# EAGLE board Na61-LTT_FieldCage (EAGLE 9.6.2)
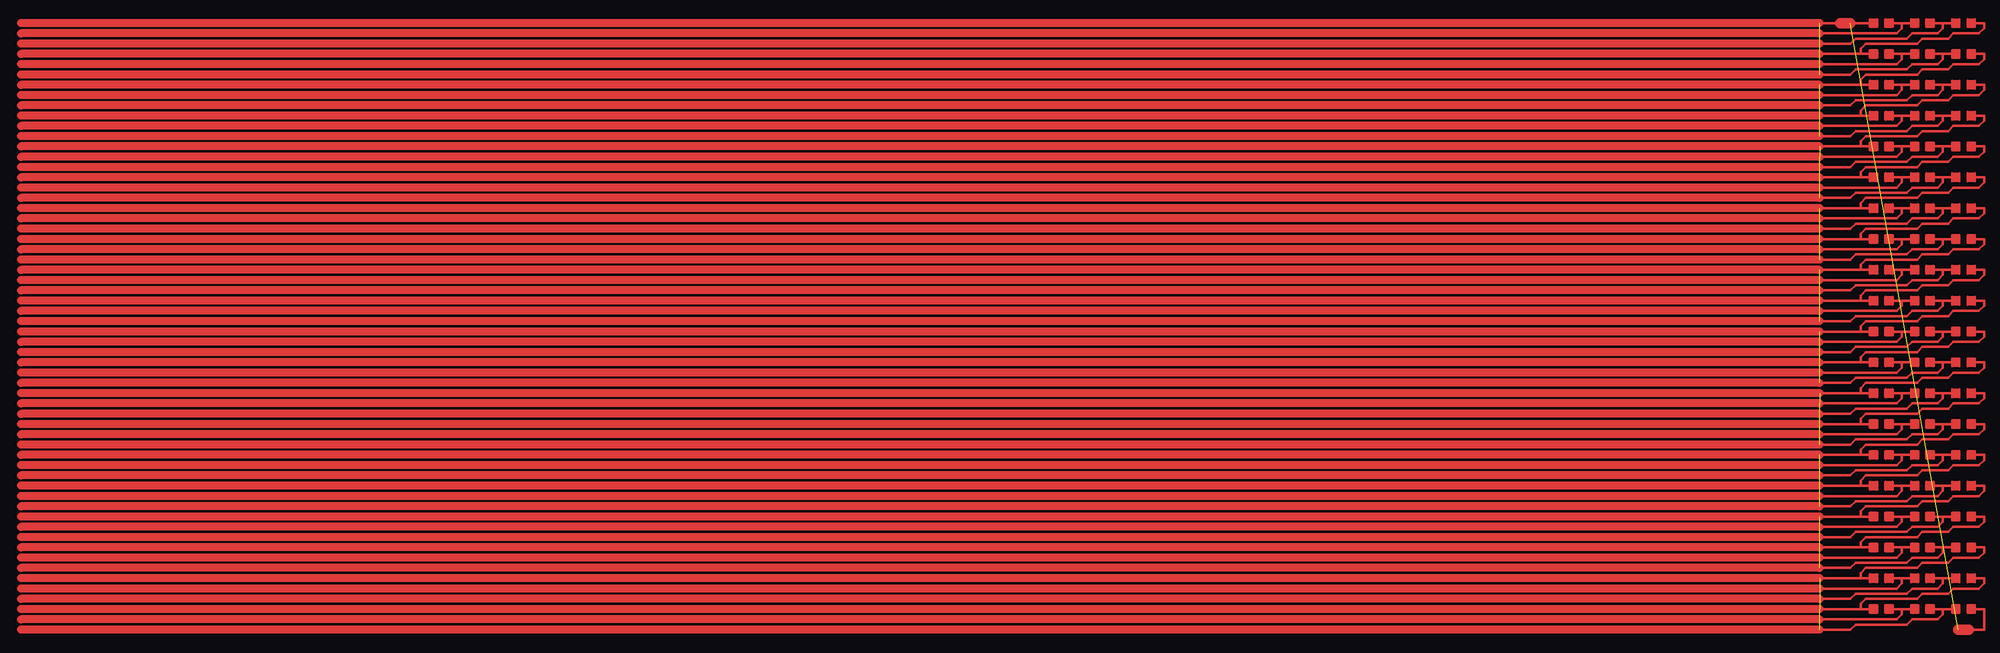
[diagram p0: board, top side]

No outline drawn. Coordinates in mm, seen from the top.
Copper layers (1*16): Top 0.035mm / dielectric 1.5mm / Bottom 0.035mm
Design rules "default": minimum track width 10mil, minimum drill 24mil, track to track 8mil, track to pad 8mil, pad to pad 8mil, via to via 8mil, smd to smd 8mil, copper to edge 40mil, drill to drill 8mil, minimum pad ring 10mil, minimum via ring 8mil, stop-mask expansion 4mil, vias tented up to drill 0mil, thermal gap 10mil

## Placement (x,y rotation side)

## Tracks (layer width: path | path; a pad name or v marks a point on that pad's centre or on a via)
S$1  (5 unrouted)
  Top 1.6: 0,2 -350,2 | 0,4 -350,4 | 0,6 -350,6 | 0,8 -350,8 | 0,10 -350,10 | 0,12 -350,12
S$2
  Top 0.406: 9.8,23.2 9.8,24.8 11.2,24.8 11.2,23.2 9.8,23.2
S$3
  Top 0.406: 12.8,23.2 12.8,24.8 14.2,24.8 14.2,23.2 12.8,23.2
S$4
  Top 0.406: 17.8,23.2 17.8,24.8 19.2,24.8 19.2,23.2 17.8,23.2
S$5
  Top 0.406: 20.8,23.2 20.8,24.8 22.2,24.8 22.2,23.2 20.8,23.2
S$6
  Top 0.406: 25.8,23.2 25.8,24.8 27.2,24.8 27.2,23.2 25.8,23.2
S$7
  Top 0.406: 28.8,23.2 28.8,24.8 30.2,24.8 30.2,23.2 28.8,23.2
S$8
  Top 0.508: 10,24 0,24
S$9
  Top 0.508: 14,24 16,24 | 16,24 18,24 | 16,24 16,23 15,22 0,22
S$10
  Top 0.508: 22,24 24,24 | 24,24 26,24 | 24,24 24,23 23,22 18,22 17,21 7,21 6,20 0,20
S$11
  Top 0.508: 8,18 8,19 9,20 19,20 20,21 25,21 26,22 31,22 32,23 32,24 30,24
S$12
  Top 0.406: 9.8,17.2 9.8,18.8 11.2,18.8 11.2,17.2 9.8,17.2
S$13
  Top 0.406: 12.8,17.2 12.8,18.8 14.2,18.8 14.2,17.2 12.8,17.2
S$14
  Top 0.406: 17.8,17.2 17.8,18.8 19.2,18.8 19.2,17.2 17.8,17.2
S$15
  Top 0.406: 9.8,5.2 9.8,6.8 11.2,6.8 11.2,5.2 9.8,5.2
S$16
  Top 0.406: 9.8,11.2 9.8,12.8 11.2,12.8 11.2,11.2 9.8,11.2
S$17
  Top 0.406: 12.8,11.2 12.8,12.8 14.2,12.8 14.2,11.2 12.8,11.2
S$18
  Top 0.406: 12.8,5.2 12.8,6.8 14.2,6.8 14.2,5.2 12.8,5.2
S$19
  Top 0.406: 17.8,11.2 17.8,12.8 19.2,12.8 19.2,11.2 17.8,11.2
S$20
  Top 0.406: 20.8,11.2 20.8,12.8 22.2,12.8 22.2,11.2 20.8,11.2
S$21
  Top 0.406: 25.8,11.2 25.8,12.8 27.2,12.8 27.2,11.2 25.8,11.2
S$22
  Top 0.406: 28.8,11.2 28.8,12.8 30.2,12.8 30.2,11.2 28.8,11.2
S$23
  Top 0.508: 8,6 8,7 9,8 19,8 20,9 25,9 26,10 31,10 32,11 32,12 30,12
S$24
  Top 0.406: 17.8,5.2 17.8,6.8 19.2,6.8 19.2,5.2 17.8,5.2
S$25
  Top 0.406: 20.8,5.2 20.8,6.8 22.2,6.8 22.2,5.2 20.8,5.2
S$26
  Top 0.508: 10,12 0,12
S$27
  Top 0.508: 14,12 16,12 | 16,12 18,12 | 16,12 16,11 15,10 0,10
S$28
  Top 0.508: 22,12 24,12 | 24,12 26,12 | 24,12 24,11 23,10 18,10 17,9 7,9 6,8 0,8
S$29
  Top 0.406: 25.8,5.2 25.8,6.8 27.2,6.8 27.2,5.2 25.8,5.2
S$30
  Top 0.406: 28.8,5.2 28.8,6.8 30.2,6.8 30.2,5.2 28.8,5.2
S$31
  Top 0.508: 10,6 0,6
S$32
  Top 0.508: 14,6 16,6 | 16,6 18,6 | 16,6 16,5 15,4 0,4
S$33
  Top 0.508: 22,6 24,6 | 24,6 26,6 | 24,6 24,5 23,4 18,4 17,3 7,3 6,2 0,2
S$34
  Top 0.508: 29,2 32,2 32,6 30,6
S$35
  Top 0.406: 20.8,17.2 20.8,18.8 22.2,18.8 22.2,17.2 20.8,17.2
S$36
  Top 0.406: 25.8,17.2 25.8,18.8 27.2,18.8 27.2,17.2 25.8,17.2
S$37
  Top 0.406: 28.8,17.2 28.8,18.8 30.2,18.8 30.2,17.2 28.8,17.2
S$38
  Top 0.508: 10,18 0,18
S$39
  Top 0.508: 14,18 16,18 | 16,18 18,18 | 16,18 16,17 15,16 0,16
S$40
  Top 0.508: 22,18 24,18 | 24,18 26,18 | 24,18 24,17 23,16 18,16 17,15 7,15 6,14 0,14
S$41
  Top 0.508: 8,12 8,13 9,14 19,14 20,15 25,15 26,16 31,16 32,17 32,18 30,18
S$42  (5 unrouted)
  Top 1.6: 0,14 -350,14 | 0,16 -350,16 | 0,18 -350,18 | 0,20 -350,20 | 0,22 -350,22 | 0,24 -350,24
S$43
  Top 0.406: 9.8,35.2 9.8,36.8 11.2,36.8 11.2,35.2 9.8,35.2
S$44
  Top 0.406: 12.8,35.2 12.8,36.8 14.2,36.8 14.2,35.2 12.8,35.2
S$45
  Top 0.406: 17.8,35.2 17.8,36.8 19.2,36.8 19.2,35.2 17.8,35.2
S$46
  Top 0.406: 20.8,35.2 20.8,36.8 22.2,36.8 22.2,35.2 20.8,35.2
S$47
  Top 0.406: 25.8,35.2 25.8,36.8 27.2,36.8 27.2,35.2 25.8,35.2
S$48
  Top 0.406: 28.8,35.2 28.8,36.8 30.2,36.8 30.2,35.2 28.8,35.2
S$49
  Top 0.508: 10,36 0,36
S$50
  Top 0.508: 14,36 16,36 | 16,36 18,36 | 16,36 16,35 15,34 0,34
S$51
  Top 0.508: 22,36 24,36 | 24,36 26,36 | 24,36 24,35 23,34 18,34 17,33 7,33 6,32 0,32
S$52
  Top 0.508: 8,30 8,31 9,32 19,32 20,33 25,33 26,34 31,34 32,35 32,36 30,36
S$53
  Top 0.406: 9.8,29.2 9.8,30.8 11.2,30.8 11.2,29.2 9.8,29.2
S$54
  Top 0.406: 12.8,29.2 12.8,30.8 14.2,30.8 14.2,29.2 12.8,29.2
S$55
  Top 0.406: 17.8,29.2 17.8,30.8 19.2,30.8 19.2,29.2 17.8,29.2
S$56
  Top 0.406: 20.8,29.2 20.8,30.8 22.2,30.8 22.2,29.2 20.8,29.2
S$57
  Top 0.406: 25.8,29.2 25.8,30.8 27.2,30.8 27.2,29.2 25.8,29.2
S$58
  Top 0.406: 28.8,29.2 28.8,30.8 30.2,30.8 30.2,29.2 28.8,29.2
S$59
  Top 0.508: 10,30 0,30
S$60
  Top 0.508: 14,30 16,30 | 16,30 18,30 | 16,30 16,29 15,28 0,28
S$61
  Top 0.508: 22,30 24,30 | 24,30 26,30 | 24,30 24,29 23,28 18,28 17,27 7,27 6,26 0,26
S$62
  Top 0.508: 8,24 8,25 9,26 19,26 20,27 25,27 26,28 31,28 32,29 32,30 30,30
S$63  (5 unrouted)
  Top 1.6: 0,26 -350,26 | 0,28 -350,28 | 0,30 -350,30 | 0,32 -350,32 | 0,34 -350,34 | 0,36 -350,36
S$64
  Top 0.406: 9.8,47.2 9.8,48.8 11.2,48.8 11.2,47.2 9.8,47.2
S$65
  Top 0.406: 12.8,47.2 12.8,48.8 14.2,48.8 14.2,47.2 12.8,47.2
S$66
  Top 0.406: 17.8,47.2 17.8,48.8 19.2,48.8 19.2,47.2 17.8,47.2
S$67
  Top 0.406: 20.8,47.2 20.8,48.8 22.2,48.8 22.2,47.2 20.8,47.2
S$68
  Top 0.406: 25.8,47.2 25.8,48.8 27.2,48.8 27.2,47.2 25.8,47.2
S$69
  Top 0.406: 28.8,47.2 28.8,48.8 30.2,48.8 30.2,47.2 28.8,47.2
S$70
  Top 0.508: 10,48 0,48
S$71
  Top 0.508: 14,48 16,48 | 16,48 18,48 | 16,48 16,47 15,46 0,46
S$72
  Top 0.508: 22,48 24,48 | 24,48 26,48 | 24,48 24,47 23,46 18,46 17,45 7,45 6,44 0,44
S$73
  Top 0.508: 8,42 8,43 9,44 19,44 20,45 25,45 26,46 31,46 32,47 32,48 30,48
S$74
  Top 0.406: 9.8,41.2 9.8,42.8 11.2,42.8 11.2,41.2 9.8,41.2
S$75
  Top 0.406: 12.8,41.2 12.8,42.8 14.2,42.8 14.2,41.2 12.8,41.2
S$76
  Top 0.406: 17.8,41.2 17.8,42.8 19.2,42.8 19.2,41.2 17.8,41.2
S$77
  Top 0.406: 20.8,41.2 20.8,42.8 22.2,42.8 22.2,41.2 20.8,41.2
S$78
  Top 0.406: 25.8,41.2 25.8,42.8 27.2,42.8 27.2,41.2 25.8,41.2
S$79
  Top 0.406: 28.8,41.2 28.8,42.8 30.2,42.8 30.2,41.2 28.8,41.2
S$80
  Top 0.508: 10,42 0,42
S$81
  Top 0.508: 14,42 16,42 | 16,42 18,42 | 16,42 16,41 15,40 0,40
S$82
  Top 0.508: 22,42 24,42 | 24,42 26,42 | 24,42 24,41 23,40 18,40 17,39 7,39 6,38 0,38
S$83
  Top 0.508: 8,36 8,37 9,38 19,38 20,39 25,39 26,40 31,40 32,41 32,42 30,42
S$84  (5 unrouted)
  Top 1.6: 0,38 -350,38 | 0,40 -350,40 | 0,42 -350,42 | 0,44 -350,44 | 0,46 -350,46 | 0,48 -350,48
S$85
  Top 0.406: 9.8,59.2 9.8,60.8 11.2,60.8 11.2,59.2 9.8,59.2
S$86
  Top 0.406: 12.8,59.2 12.8,60.8 14.2,60.8 14.2,59.2 12.8,59.2
S$87
  Top 0.406: 17.8,59.2 17.8,60.8 19.2,60.8 19.2,59.2 17.8,59.2
S$88
  Top 0.406: 20.8,59.2 20.8,60.8 22.2,60.8 22.2,59.2 20.8,59.2
S$89
  Top 0.406: 25.8,59.2 25.8,60.8 27.2,60.8 27.2,59.2 25.8,59.2
S$90
  Top 0.406: 28.8,59.2 28.8,60.8 30.2,60.8 30.2,59.2 28.8,59.2
S$91
  Top 0.508: 10,60 0,60
S$92
  Top 0.508: 14,60 16,60 | 16,60 18,60 | 16,60 16,59 15,58 0,58
S$93
  Top 0.508: 22,60 24,60 | 24,60 26,60 | 24,60 24,59 23,58 18,58 17,57 7,57 6,56 0,56
S$94
  Top 0.508: 8,54 8,55 9,56 19,56 20,57 25,57 26,58 31,58 32,59 32,60 30,60
S$95
  Top 0.406: 9.8,53.2 9.8,54.8 11.2,54.8 11.2,53.2 9.8,53.2
S$96
  Top 0.406: 12.8,53.2 12.8,54.8 14.2,54.8 14.2,53.2 12.8,53.2
S$97
  Top 0.406: 17.8,53.2 17.8,54.8 19.2,54.8 19.2,53.2 17.8,53.2
S$98
  Top 0.406: 20.8,53.2 20.8,54.8 22.2,54.8 22.2,53.2 20.8,53.2
S$99
  Top 0.406: 25.8,53.2 25.8,54.8 27.2,54.8 27.2,53.2 25.8,53.2
S$100
  Top 0.406: 28.8,53.2 28.8,54.8 30.2,54.8 30.2,53.2 28.8,53.2
S$101
  Top 0.508: 10,54 0,54
S$102
  Top 0.508: 14,54 16,54 | 16,54 18,54 | 16,54 16,53 15,52 0,52
S$103
  Top 0.508: 22,54 24,54 | 24,54 26,54 | 24,54 24,53 23,52 18,52 17,51 7,51 6,50 0,50
S$104
  Top 0.508: 8,48 8,49 9,50 19,50 20,51 25,51 26,52 31,52 32,53 32,54 30,54
S$105  (5 unrouted)
  Top 1.6: 0,50 -350,50 | 0,52 -350,52 | 0,54 -350,54 | 0,56 -350,56 | 0,58 -350,58 | 0,60 -350,60
S$106
  Top 0.406: 9.8,71.2 9.8,72.8 11.2,72.8 11.2,71.2 9.8,71.2
S$107
  Top 0.406: 12.8,71.2 12.8,72.8 14.2,72.8 14.2,71.2 12.8,71.2
S$108
  Top 0.406: 17.8,71.2 17.8,72.8 19.2,72.8 19.2,71.2 17.8,71.2
S$109
  Top 0.406: 20.8,71.2 20.8,72.8 22.2,72.8 22.2,71.2 20.8,71.2
S$110
  Top 0.406: 25.8,71.2 25.8,72.8 27.2,72.8 27.2,71.2 25.8,71.2
S$111
  Top 0.406: 28.8,71.2 28.8,72.8 30.2,72.8 30.2,71.2 28.8,71.2
S$112
  Top 0.508: 10,72 0,72
S$113
  Top 0.508: 14,72 16,72 | 16,72 18,72 | 16,72 16,71 15,70 0,70
S$114
  Top 0.508: 22,72 24,72 | 24,72 26,72 | 24,72 24,71 23,70 18,70 17,69 7,69 6,68 0,68
S$115
  Top 0.508: 8,66 8,67 9,68 19,68 20,69 25,69 26,70 31,70 32,71 32,72 30,72
S$116
  Top 0.406: 9.8,65.2 9.8,66.8 11.2,66.8 11.2,65.2 9.8,65.2
S$117
  Top 0.406: 12.8,65.2 12.8,66.8 14.2,66.8 14.2,65.2 12.8,65.2
S$118
  Top 0.406: 17.8,65.2 17.8,66.8 19.2,66.8 19.2,65.2 17.8,65.2
S$119
  Top 0.406: 20.8,65.2 20.8,66.8 22.2,66.8 22.2,65.2 20.8,65.2
S$120
  Top 0.406: 25.8,65.2 25.8,66.8 27.2,66.8 27.2,65.2 25.8,65.2
S$121
  Top 0.406: 28.8,65.2 28.8,66.8 30.2,66.8 30.2,65.2 28.8,65.2
S$122
  Top 0.508: 10,66 0,66
S$123
  Top 0.508: 14,66 16,66 | 16,66 18,66 | 16,66 16,65 15,64 0,64
S$124
  Top 0.508: 22,66 24,66 | 24,66 26,66 | 24,66 24,65 23,64 18,64 17,63 7,63 6,62 0,62
S$125
  Top 0.508: 8,60 8,61 9,62 19,62 20,63 25,63 26,64 31,64 32,65 32,66 30,66
S$126  (5 unrouted)
  Top 1.6: 0,62 -350,62 | 0,64 -350,64 | 0,66 -350,66 | 0,68 -350,68 | 0,70 -350,70 | 0,72 -350,72
S$127
  Top 0.406: 9.8,83.2 9.8,84.8 11.2,84.8 11.2,83.2 9.8,83.2
S$128
  Top 0.406: 12.8,83.2 12.8,84.8 14.2,84.8 14.2,83.2 12.8,83.2
S$129
  Top 0.406: 17.8,83.2 17.8,84.8 19.2,84.8 19.2,83.2 17.8,83.2
S$130
  Top 0.406: 20.8,83.2 20.8,84.8 22.2,84.8 22.2,83.2 20.8,83.2
S$131
  Top 0.406: 25.8,83.2 25.8,84.8 27.2,84.8 27.2,83.2 25.8,83.2
S$132
  Top 0.406: 28.8,83.2 28.8,84.8 30.2,84.8 30.2,83.2 28.8,83.2
S$133
  Top 0.508: 10,84 0,84
S$134
  Top 0.508: 14,84 16,84 | 16,84 18,84 | 16,84 16,83 15,82 0,82
S$135
  Top 0.508: 22,84 24,84 | 24,84 26,84 | 24,84 24,83 23,82 18,82 17,81 7,81 6,80 0,80
S$136
  Top 0.508: 8,78 8,79 9,80 19,80 20,81 25,81 26,82 31,82 32,83 32,84 30,84
S$137
  Top 0.406: 9.8,77.2 9.8,78.8 11.2,78.8 11.2,77.2 9.8,77.2
S$138
  Top 0.406: 12.8,77.2 12.8,78.8 14.2,78.8 14.2,77.2 12.8,77.2
S$139
  Top 0.406: 17.8,77.2 17.8,78.8 19.2,78.8 19.2,77.2 17.8,77.2
S$140
  Top 0.406: 20.8,77.2 20.8,78.8 22.2,78.8 22.2,77.2 20.8,77.2
S$141
  Top 0.406: 25.8,77.2 25.8,78.8 27.2,78.8 27.2,77.2 25.8,77.2
S$142
  Top 0.406: 28.8,77.2 28.8,78.8 30.2,78.8 30.2,77.2 28.8,77.2
S$143
  Top 0.508: 10,78 0,78
S$144
  Top 0.508: 14,78 16,78 | 16,78 18,78 | 16,78 16,77 15,76 0,76
S$145
  Top 0.508: 22,78 24,78 | 24,78 26,78 | 24,78 24,77 23,76 18,76 17,75 7,75 6,74 0,74
S$146
  Top 0.508: 8,72 8,73 9,74 19,74 20,75 25,75 26,76 31,76 32,77 32,78 30,78
S$147  (5 unrouted)
  Top 1.6: 0,74 -350,74 | 0,76 -350,76 | 0,78 -350,78 | 0,80 -350,80 | 0,82 -350,82 | 0,84 -350,84
S$148
  Top 0.406: 9.8,95.2 9.8,96.8 11.2,96.8 11.2,95.2 9.8,95.2
S$149
  Top 0.406: 12.8,95.2 12.8,96.8 14.2,96.8 14.2,95.2 12.8,95.2
S$150
  Top 0.406: 17.8,95.2 17.8,96.8 19.2,96.8 19.2,95.2 17.8,95.2
S$151
  Top 0.406: 20.8,95.2 20.8,96.8 22.2,96.8 22.2,95.2 20.8,95.2
S$152
  Top 0.406: 25.8,95.2 25.8,96.8 27.2,96.8 27.2,95.2 25.8,95.2
S$153
  Top 0.406: 28.8,95.2 28.8,96.8 30.2,96.8 30.2,95.2 28.8,95.2
S$154
  Top 0.508: 10,96 0,96
S$155
  Top 0.508: 14,96 16,96 | 16,96 18,96 | 16,96 16,95 15,94 0,94
S$156
  Top 0.508: 22,96 24,96 | 24,96 26,96 | 24,96 24,95 23,94 18,94 17,93 7,93 6,92 0,92
S$157
  Top 0.508: 8,90 8,91 9,92 19,92 20,93 25,93 26,94 31,94 32,95 32,96 30,96
S$158
  Top 0.406: 9.8,89.2 9.8,90.8 11.2,90.8 11.2,89.2 9.8,89.2
S$159
  Top 0.406: 12.8,89.2 12.8,90.8 14.2,90.8 14.2,89.2 12.8,89.2
S$160
  Top 0.406: 17.8,89.2 17.8,90.8 19.2,90.8 19.2,89.2 17.8,89.2
S$161
  Top 0.406: 20.8,89.2 20.8,90.8 22.2,90.8 22.2,89.2 20.8,89.2
S$162
  Top 0.406: 25.8,89.2 25.8,90.8 27.2,90.8 27.2,89.2 25.8,89.2
S$163
  Top 0.406: 28.8,89.2 28.8,90.8 30.2,90.8 30.2,89.2 28.8,89.2
S$164
  Top 0.508: 10,90 0,90
S$165
  Top 0.508: 14,90 16,90 | 16,90 18,90 | 16,90 16,89 15,88 0,88
S$166
  Top 0.508: 22,90 24,90 | 24,90 26,90 | 24,90 24,89 23,88 18,88 17,87 7,87 6,86 0,86
S$167
  Top 0.508: 8,84 8,85 9,86 19,86 20,87 25,87 26,88 31,88 32,89 32,90 30,90
S$168  (5 unrouted)
  Top 1.6: 0,86 -350,86 | 0,88 -350,88 | 0,90 -350,90 | 0,92 -350,92 | 0,94 -350,94 | 0,96 -350,96
S$169
  Top 0.406: 9.8,107.2 9.8,108.8 11.2,108.8 11.2,107.2 9.8,107.2
S$170
  Top 0.406: 12.8,107.2 12.8,108.8 14.2,108.8 14.2,107.2 12.8,107.2
S$171
  Top 0.406: 17.8,107.2 17.8,108.8 19.2,108.8 19.2,107.2 17.8,107.2
S$172
  Top 0.406: 20.8,107.2 20.8,108.8 22.2,108.8 22.2,107.2 20.8,107.2
S$173
  Top 0.406: 25.8,107.2 25.8,108.8 27.2,108.8 27.2,107.2 25.8,107.2
S$174
  Top 0.406: 28.8,107.2 28.8,108.8 30.2,108.8 30.2,107.2 28.8,107.2
S$175
  Top 0.508: 10,108 0,108
S$176
  Top 0.508: 14,108 16,108 | 16,108 18,108 | 16,108 16,107 15,106 0,106
S$177
  Top 0.508: 22,108 24,108 | 24,108 26,108 | 24,108 24,107 23,106 18,106 17,105 7,105 6,104 0,104
S$178
  Top 0.508: 8,102 8,103 9,104 19,104 20,105 25,105 26,106 31,106 32,107 32,108 30,108
S$179
  Top 0.406: 9.8,101.2 9.8,102.8 11.2,102.8 11.2,101.2 9.8,101.2
S$180
  Top 0.406: 12.8,101.2 12.8,102.8 14.2,102.8 14.2,101.2 12.8,101.2
S$181
  Top 0.406: 17.8,101.2 17.8,102.8 19.2,102.8 19.2,101.2 17.8,101.2
S$182
  Top 0.406: 20.8,101.2 20.8,102.8 22.2,102.8 22.2,101.2 20.8,101.2
S$183
  Top 0.406: 25.8,101.2 25.8,102.8 27.2,102.8 27.2,101.2 25.8,101.2
S$184
  Top 0.406: 28.8,101.2 28.8,102.8 30.2,102.8 30.2,101.2 28.8,101.2
S$185
  Top 0.508: 10,102 0,102
S$186
  Top 0.508: 14,102 16,102 | 16,102 18,102 | 16,102 16,101 15,100 0,100
S$187
  Top 0.508: 22,102 24,102 | 24,102 26,102 | 24,102 24,101 23,100 18,100 17,99 7,99 6,98 0,98
S$188
  Top 0.508: 8,96 8,97 9,98 19,98 20,99 25,99 26,100 31,100 32,101 32,102 30,102
S$189  (5 unrouted)
  Top 1.6: 0,98 -350,98 | 0,100 -350,100 | 0,102 -350,102 | 0,104 -350,104 | 0,106 -350,106 | 0,108 -350,108
S$190
  Top 0.406: 9.8,119.2 9.8,120.8 11.2,120.8 11.2,119.2 9.8,119.2
S$191
  Top 0.406: 12.8,119.2 12.8,120.8 14.2,120.8 14.2,119.2 12.8,119.2
S$192
  Top 0.406: 17.8,119.2 17.8,120.8 19.2,120.8 19.2,119.2 17.8,119.2
S$193
  Top 0.406: 20.8,119.2 20.8,120.8 22.2,120.8 22.2,119.2 20.8,119.2
S$194
  Top 0.406: 25.8,119.2 25.8,120.8 27.2,120.8 27.2,119.2 25.8,119.2
S$195
  Top 0.406: 28.8,119.2 28.8,120.8 30.2,120.8 30.2,119.2 28.8,119.2
S$196
  Top 0.508: 10,120 0,120
S$197
  Top 0.508: 14,120 16,120 | 16,120 18,120 | 16,120 16,119 15,118 0,118
S$198
  Top 0.508: 22,120 24,120 | 24,120 26,120 | 24,120 24,119 23,118 18,118 17,117 7,117 6,116 0,116
S$199
  Top 0.508: 8,114 8,115 9,116 19,116 20,117 25,117 26,118 31,118 32,119 32,120 30,120
S$200
  Top 0.406: 9.8,113.2 9.8,114.8 11.2,114.8 11.2,113.2 9.8,113.2
S$201
  Top 0.406: 12.8,113.2 12.8,114.8 14.2,114.8 14.2,113.2 12.8,113.2
S$202
  Top 0.406: 17.8,113.2 17.8,114.8 19.2,114.8 19.2,113.2 17.8,113.2
S$203
  Top 0.406: 20.8,113.2 20.8,114.8 22.2,114.8 22.2,113.2 20.8,113.2
S$204
  Top 0.406: 25.8,113.2 25.8,114.8 27.2,114.8 27.2,113.2 25.8,113.2
S$205
  Top 0.406: 28.8,113.2 28.8,114.8 30.2,114.8 30.2,113.2 28.8,113.2
S$206
  Top 0.508: 10,114 0,114
S$207
  Top 0.508: 14,114 16,114 | 16,114 18,114 | 16,114 16,113 15,112 0,112
S$208
  Top 0.508: 22,114 24,114 | 24,114 26,114 | 24,114 24,113 23,112 18,112 17,111 7,111 6,110 0,110
S$209
  Top 0.508: 8,108 8,109 9,110 19,110 20,111 25,111 26,112 31,112 32,113 32,114 30,114
S$210  (5 unrouted)
  Top 1.6: 0,110 -350,110 | 0,112 -350,112 | 0,114 -350,114 | 0,116 -350,116 | 0,118 -350,118 | 0,120 -350,120
S$253  (1 unrouted)
  Top 2: 4,120 6,120 | 27,2 29,2
(copper drawn outside any net)
  shapes: Top area x120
